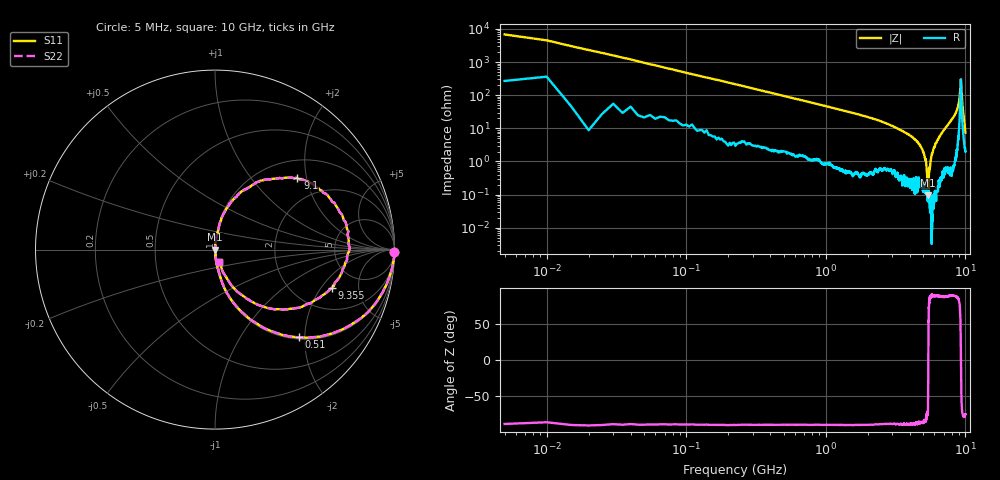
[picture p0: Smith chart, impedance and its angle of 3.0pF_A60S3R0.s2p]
! Amotech Co.,Ltd.
! http://www.amotech.co.kr/
! Part Number: A60S3R0
! These Parameters are Measured in Series Mode Connection
! Operation Temp=25[degC], DC Bias Voltage=0[V]
! Freq. Start=5[MHz] Stop=10[GHz], 2000[Steps]
! Date: Monday, July 13, 2020, 01:26:55
# GHZ S RI R 50.000000
!Freq.(Hz) S11(Real) S11(Imag) S21(Real) S21(Imag) S12(Real) S12(Imag) S22(Real) S22(Imag)
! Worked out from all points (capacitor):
!   2000 points, 5 MHz to 10 GHz, reference 50 ohm
!   read as one part in series: C = 3.35 pF near 55 MHz
!   lowest |Z| = 96.3 mohm at 5.42 GHz (marker M1)
!   series resonance near 5.427 GHz, so ESL is about 260 pH
!   S11 on the Smith chart (normalised r, x): 5 MHz: open; 510 MHz: 1.04, -1.88; 9.1 GHz: 1.40, +1.76; 9.355 GHz: 3.16, -2.54; 10 GHz: 1.04, -0.14
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0.005  0.9992 -0.0147  0.000796 0.0147  0.000796 0.0147  0.9992 -0.0147
0.075  0.9717 -0.1524  0.0283 0.1524  0.0283 0.1524  0.9717 -0.1524
0.145  0.9118 -0.2742  0.0882 0.2742  0.0882 0.2742  0.9118 -0.2742
0.51  0.4697 -0.4886  0.5303 0.4886  0.5303 0.4886  0.4697 -0.4886
0.955  0.1988 -0.391  0.8012 0.391  0.8012 0.391  0.1988 -0.391
1.675  0.0712 -0.2486  0.9288 0.2486  0.9288 0.2486  0.0712 -0.2486
3.34  0.0117 -0.0924  0.9883 0.0924  0.9883 0.0924  0.0117 -0.0924
4.385  0.00413 -0.0453  0.9959 0.0453  0.9959 0.0453  0.00413 -0.0453
5.005  0.00163 -0.0189  0.9984 0.0189  0.9984 0.0189  0.00163 -0.0189
5.22  0.00138 -0.0101  0.9986 0.0101  0.9986 0.0101  0.00138 -0.0101
5.42  0.000895 -0.000353  0.9991 0.000353  0.9991 0.000353  0.000895 -0.000353
5.52  0.000903 0.00538  0.9991 -0.00538  0.9991 -0.00538  0.000903 0.00538
5.735  0.000284 0.0159  0.9997 -0.0159  0.9997 -0.0159  0.000284 0.0159
6.67  0.00738 0.0642  0.9926 -0.0642  0.9926 -0.0642  0.00738 0.0642
8.335  0.0619 0.2258  0.9381 -0.2258  0.9381 -0.2258  0.0619 0.2258
8.835  0.1791 0.3403  0.8209 -0.3403  0.8209 -0.3403  0.1791 0.3403
9.1  0.459 0.3973  0.541 -0.3973  0.541 -0.3973  0.459 0.3973
9.27  0.7427 0.0663  0.2573 -0.0663  0.2573 -0.0663  0.7427 0.0663
9.355  0.6496 -0.2138  0.3504 0.2138  0.3504 0.2138  0.6496 -0.2138
9.455  0.3983 -0.3335  0.6017 0.3335  0.6017 0.3335  0.3983 -0.3335
9.61  0.1578 -0.2595  0.8422 0.2595  0.8422 0.2595  0.1578 -0.2595
10  0.0242 -0.0683  0.9758 0.0683  0.9758 0.0683  0.0242 -0.0683
